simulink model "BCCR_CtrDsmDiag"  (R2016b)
settings: Solver=FixedStepDiscrete  StartTime=0.0  StopTime=10.0  FixedStep=0.02  RelTol=1e-3  EnableMultiTasking=on
undefined symbols (not defined in the file or in its folder): BCCR_cntDChrgCtrPlausDiag_CW, BCCR_cntMainCtrPlausDiag_CW, bin2dec
libraries: simulink x72

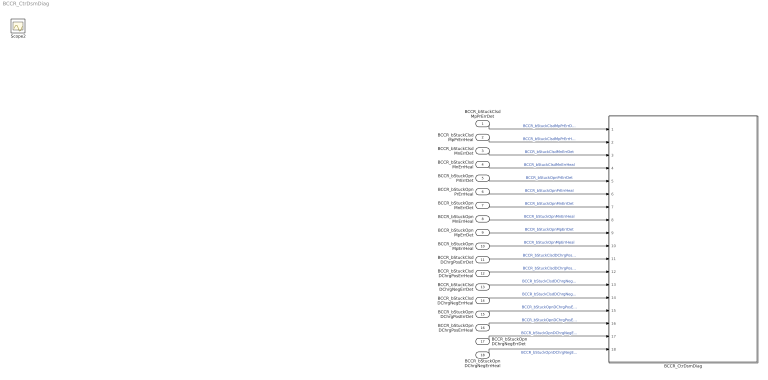
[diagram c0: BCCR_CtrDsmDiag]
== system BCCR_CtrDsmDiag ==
  BCCR_bStuckClsdMpPrErrDet : Inport
  BCCR_bStuckClsdMpPrErrHeal : Inport  Port=2
  BCCR_bStuckClsdMnErrDet : Inport  Port=3
  BCCR_bStuckClsdMnErrHeal : Inport  Port=4
  BCCR_bStuckOpnPrErrDet : Inport  Port=5
  BCCR_bStuckOpnPrErrHeal : Inport  Port=6
  BCCR_bStuckOpnMnErrDet : Inport  Port=7
  BCCR_bStuckOpnMnErrHeal : Inport  Port=8
  BCCR_bStuckOpnMpErrDet : Inport  Port=9
  BCCR_bStuckOpnMpErrHeal : Inport  Port=10
  BCCR_bStuckClsdDChrgPosErrDet : Inport  Port=11
  BCCR_bStuckClsdDChrgPosErrHeal : Inport  Port=12
  BCCR_bStuckClsdDChrgNegErrDet : Inport  Port=13
  BCCR_bStuckClsdDChrgNegErrHeal : Inport  Port=14
  BCCR_bStuckOpnDChrgPosErrDet : Inport  Port=15
  BCCR_bStuckOpnDChrgPosErrHeal : Inport  Port=16
  BCCR_bStuckOpnDChrgNegErrDet : Inport  Port=17
  BCCR_bStuckOpnDChrgNegErrHeal : Inport  Port=18
  BCCR_CtrDsmDiag : Subsystem
  Scope2 : Scope
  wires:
  BCCR_bStuckClsdMpPrErrDet/1 -> BCCR_CtrDsmDiag/1(BCCR_bStuckClsdMpPrErrDet)  "BCCR_bStuckClsdMpPrErrDet"
  BCCR_bStuckClsdMpPrErrHeal/1 -> BCCR_CtrDsmDiag/2(BCCR_bStuckClsdMpPrErrHeal)  "BCCR_bStuckClsdMpPrErrHeal"
  BCCR_bStuckClsdMnErrDet/1 -> BCCR_CtrDsmDiag/3(BCCR_bStuckClsdMnErrDet)  "BCCR_bStuckClsdMnErrDet"
  BCCR_bStuckClsdMnErrHeal/1 -> BCCR_CtrDsmDiag/4(BCCR_bStuckClsdMnErrHeal)  "BCCR_bStuckClsdMnErrHeal"
  BCCR_bStuckOpnPrErrDet/1 -> BCCR_CtrDsmDiag/5(BCCR_bStuckOpnPrErrDet)  "BCCR_bStuckOpnPrErrDet"
  BCCR_bStuckOpnPrErrHeal/1 -> BCCR_CtrDsmDiag/6(BCCR_bStuckOpnPrErrHeal)  "BCCR_bStuckOpnPrErrHeal"
  BCCR_bStuckOpnMnErrDet/1 -> BCCR_CtrDsmDiag/7(BCCR_bStuckOpnMnErrDet)  "BCCR_bStuckOpnMnErrDet"
  BCCR_bStuckOpnMnErrHeal/1 -> BCCR_CtrDsmDiag/8(BCCR_bStuckOpnMnErrHeal)  "BCCR_bStuckOpnMnErrHeal"
  BCCR_bStuckOpnMpErrDet/1 -> BCCR_CtrDsmDiag/9(BCCR_bStuckOpnMpErrDet)  "BCCR_bStuckOpnMpErrDet"
  BCCR_bStuckOpnMpErrHeal/1 -> BCCR_CtrDsmDiag/10(BCCR_bStuckOpnMpErrHeal)  "BCCR_bStuckOpnMpErrHeal"
  BCCR_bStuckClsdDChrgPosErrDet/1 -> BCCR_CtrDsmDiag/11(BCCR_bStuckClsdDChrgPosErrDet)  "BCCR_bStuckClsdDChrgPosErrDet"
  BCCR_bStuckClsdDChrgPosErrHeal/1 -> BCCR_CtrDsmDiag/12(BCCR_bStuckClsdDChrgPosErrHeal)  "BCCR_bStuckClsdDChrgPosErrHeal"
  BCCR_bStuckClsdDChrgNegErrDet/1 -> BCCR_CtrDsmDiag/13(BCCR_bStuckClsdDChrgNegErrDet)  "BCCR_bStuckClsdDChrgNegErrDet"
  BCCR_bStuckClsdDChrgNegErrHeal/1 -> BCCR_CtrDsmDiag/14(BCCR_bStuckClsdDChrgNegErrHeal)  "BCCR_bStuckClsdDChrgNegErrHeal"
  BCCR_bStuckOpnDChrgPosErrDet/1 -> BCCR_CtrDsmDiag/15(BCCR_bStuckOpnDChrgPosErrDet)  "BCCR_bStuckOpnDChrgPosErrDet"
  BCCR_bStuckOpnDChrgPosErrHeal/1 -> BCCR_CtrDsmDiag/16(BCCR_bStuckOpnDChrgPosErrHeal)  "BCCR_bStuckOpnDChrgPosErrHeal"
  BCCR_bStuckOpnDChrgNegErrDet/1 -> BCCR_CtrDsmDiag/17(BCCR_bStuckOpnDChrgNegErrDet)  "BCCR_bStuckOpnDChrgNegErrDet"
  BCCR_bStuckOpnDChrgNegErrHeal/1 -> BCCR_CtrDsmDiag/18(BCCR_bStuckOpnDChrgNegErrHeal)  "BCCR_bStuckOpnDChrgNegErrHeal"

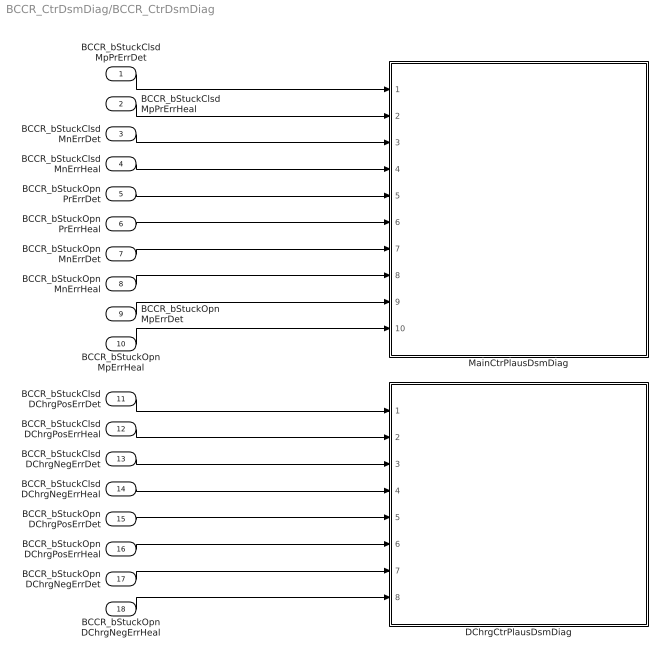
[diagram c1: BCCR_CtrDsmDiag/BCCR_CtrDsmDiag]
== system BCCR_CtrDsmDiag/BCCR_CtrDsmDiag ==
  BCCR_bStuckClsdMpPrErrDet : Inport
  BCCR_bStuckClsdMpPrErrHeal : Inport  Port=2
  BCCR_bStuckClsdMnErrDet : Inport  Port=3
  BCCR_bStuckClsdMnErrHeal : Inport  Port=4
  BCCR_bStuckOpnPrErrDet : Inport  Port=5
  BCCR_bStuckOpnPrErrHeal : Inport  Port=6
  BCCR_bStuckOpnMnErrDet : Inport  Port=7
  BCCR_bStuckOpnMnErrHeal : Inport  Port=8
  BCCR_bStuckOpnMpErrDet : Inport  Port=9
  BCCR_bStuckOpnMpErrHeal : Inport  Port=10
  BCCR_bStuckClsdDChrgPosErrDet : Inport  Port=11
  BCCR_bStuckClsdDChrgPosErrHeal : Inport  Port=12
  BCCR_bStuckClsdDChrgNegErrDet : Inport  Port=13
  BCCR_bStuckClsdDChrgNegErrHeal : Inport  Port=14
  BCCR_bStuckOpnDChrgPosErrDet : Inport  Port=15
  BCCR_bStuckOpnDChrgPosErrHeal : Inport  Port=16
  BCCR_bStuckOpnDChrgNegErrDet : Inport  Port=17
  BCCR_bStuckOpnDChrgNegErrHeal : Inport  Port=18
  DChrgCtrPlausDsmDiag : Subsystem
  MainCtrPlausDsmDiag : Subsystem
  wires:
  BCCR_bStuckClsdDChrgPosErrHeal/1 -> DChrgCtrPlausDsmDiag/2(BCCR_bStuckClsdDChrgPosErrHeal)
  BCCR_bStuckClsdDChrgNegErrHeal/1 -> DChrgCtrPlausDsmDiag/4(BCCR_bStuckClsdDChrgNegErrHeal)
  BCCR_bStuckOpnDChrgPosErrHeal/1 -> DChrgCtrPlausDsmDiag/6(BCCR_bStuckOpnDChrgPosErrHeal)
  BCCR_bStuckOpnDChrgNegErrDet/1 -> DChrgCtrPlausDsmDiag/7(BCCR_bStuckOpnDChrgNegErrDet)
  BCCR_bStuckOpnDChrgNegErrHeal/1 -> DChrgCtrPlausDsmDiag/8(BCCR_bStuckOpnDChrgNegErrHeal)
  BCCR_bStuckClsdMnErrDet/1 -> MainCtrPlausDsmDiag/3(BCCR_bStuckClsdMnErrDet)
  BCCR_bStuckClsdDChrgNegErrDet/1 -> DChrgCtrPlausDsmDiag/3(BCCR_bStuckClsdDChrgNegErrDet)
  BCCR_bStuckClsdMnErrHeal/1 -> MainCtrPlausDsmDiag/4(BCCR_bStuckClsdMnErrHeal)
  BCCR_bStuckClsdMpPrErrDet/1 -> MainCtrPlausDsmDiag/1(BCCR_bStuckClsdMpPrErrDet)
  BCCR_bStuckClsdMpPrErrHeal/1 -> MainCtrPlausDsmDiag/2(BCCR_bStuckClsdMpPrErrHeal)
  BCCR_bStuckClsdDChrgPosErrDet/1 -> DChrgCtrPlausDsmDiag/1(BCCR_bStuckClsdDChrgPosErrDet)
  BCCR_bStuckOpnDChrgPosErrDet/1 -> DChrgCtrPlausDsmDiag/5(BCCR_bStuckOpnDChrgPosErrDet)
  BCCR_bStuckOpnPrErrHeal/1 -> MainCtrPlausDsmDiag/6(BCCR_bStuckOpnPrErrHeal)
  BCCR_bStuckOpnMnErrDet/1 -> MainCtrPlausDsmDiag/7(BCCR_bStuckOpnMnErrDet)
  BCCR_bStuckOpnMpErrHeal/1 -> MainCtrPlausDsmDiag/10(BCCR_bStuckOpnMpErrHeal)
  BCCR_bStuckOpnPrErrDet/1 -> MainCtrPlausDsmDiag/5(BCCR_bStuckOpnPrErrDet)
  BCCR_bStuckOpnMpErrDet/1 -> MainCtrPlausDsmDiag/9(BCCR_bStuckOpnMpErrDet)
  BCCR_bStuckOpnMnErrHeal/1 -> MainCtrPlausDsmDiag/8(BCCR_bStuckOpnMnErrHeal)

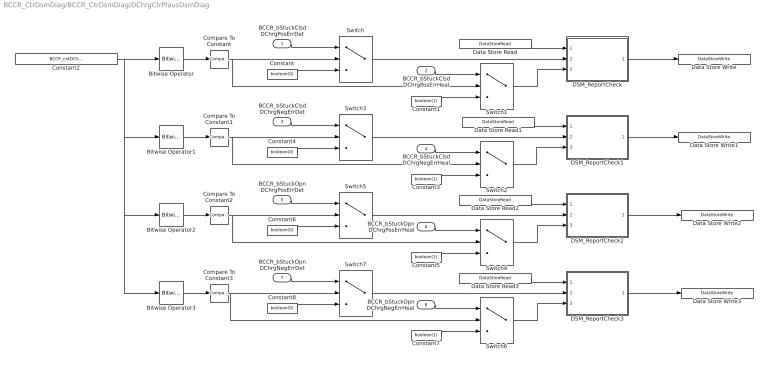
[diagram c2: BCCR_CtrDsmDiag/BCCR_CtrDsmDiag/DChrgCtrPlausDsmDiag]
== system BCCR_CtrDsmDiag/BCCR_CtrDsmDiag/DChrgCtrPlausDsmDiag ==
  BCCR_bStuckClsdDChrgPosErrDet : Inport
  BCCR_bStuckClsdDChrgPosErrHeal : Inport  Port=2
  BCCR_bStuckClsdDChrgNegErrDet : Inport  Port=3
  BCCR_bStuckClsdDChrgNegErrHeal : Inport  Port=4
  BCCR_bStuckOpnDChrgPosErrDet : Inport  Port=5
  BCCR_bStuckOpnDChrgPosErrHeal : Inport  Port=6
  BCCR_bStuckOpnDChrgNegErrDet : Inport  Port=7
  BCCR_bStuckOpnDChrgNegErrHeal : Inport  Port=8
  Bitwise Operator : simulink/Logic and Bit Operations/Bitwise Operator  logicop=AND  UseBitMask=on  BitMask=bin2dec('00000001')  BitMaskRealWorld=Stored Integer
  Bitwise Operator1 : simulink/Logic and Bit Operations/Bitwise Operator  logicop=AND  UseBitMask=on  BitMask=bin2dec('00000010')  BitMaskRealWorld=Stored Integer
  Bitwise Operator2 : simulink/Logic and Bit Operations/Bitwise Operator  logicop=AND  UseBitMask=on  BitMask=bin2dec('00000100')  BitMaskRealWorld=Stored Integer
  Bitwise Operator3 : simulink/Logic and Bit Operations/Bitwise Operator  logicop=AND  UseBitMask=on  BitMask=bin2dec('00001000')  BitMaskRealWorld=Stored Integer
  Compare To Constant : simulink/Logic and Bit Operations/Compare To Constant  relop===  const=1  OutDataTypeStr=boolean
  Compare To Constant1 : simulink/Logic and Bit Operations/Compare To Constant  relop===  const=2  OutDataTypeStr=boolean
  Compare To Constant2 : simulink/Logic and Bit Operations/Compare To Constant  relop===  const=4  OutDataTypeStr=boolean
  Compare To Constant3 : simulink/Logic and Bit Operations/Compare To Constant  relop===  const=8  OutDataTypeStr=boolean
  Constant{,4,6,8} (4 alike) : Constant  Value=boolean(0)  OutDataTypeStr=boolean
  Constant{1,3,5,7} (4 alike) : Constant  Value=boolean(1)  OutDataTypeStr=boolean
  Constant2 : Constant  Value=BCCR_cntDChrgCtrPlausDiag_CW
  DSM_ReportCheck : Subsystem  TreatAsAtomicUnit=on  RTWFcnName=DSM_ReportCheck  RTWFileName=SrvLib
  DSM_ReportCheck1 : Subsystem  TreatAsAtomicUnit=on  RTWFcnName=DSM_ReportCheck  RTWFileName=SrvLib
  DSM_ReportCheck2 : Subsystem  TreatAsAtomicUnit=on  RTWFcnName=DSM_ReportCheck  RTWFileName=SrvLib
  DSM_ReportCheck3 : Subsystem  TreatAsAtomicUnit=on  RTWFcnName=DSM_ReportCheck  RTWFileName=SrvLib
  Data Store Read : DataStoreRead  DataStoreName=DFC_DChrgPosStuckMax
  Data Store Read1 : DataStoreRead  DataStoreName=DFC_DChrgNegStuckMax
  Data Store Read2 : DataStoreRead  DataStoreName=DFC_DChrgPosStuckMin
  Data Store Read3 : DataStoreRead  DataStoreName=DFC_DChrgNegStuckMin
  Data Store Write : DataStoreWrite  DataStoreName=DFC_DChrgPosStuckMax
  Data Store Write1 : DataStoreWrite  DataStoreName=DFC_DChrgNegStuckMax
  Data Store Write2 : DataStoreWrite  DataStoreName=DFC_DChrgPosStuckMin
  Data Store Write3 : DataStoreWrite  DataStoreName=DFC_DChrgNegStuckMin
  Switch{,1..7} (8 alike) : Switch  Criteria=u2 > Threshold
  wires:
  DSM_ReportCheck/1(Dfc_id) -> Data Store Write/1
  DSM_ReportCheck1/1(Dfc_id) -> Data Store Write1/1
  Data Store Read2/1 -> DSM_ReportCheck2/1(Dfc_id_nv)
  Data Store Read/1 -> DSM_ReportCheck/1(Dfc_id_nv)
  DSM_ReportCheck2/1(Dfc_id) -> Data Store Write2/1
  Data Store Read3/1 -> DSM_ReportCheck3/1(Dfc_id_nv)
  Data Store Read1/1 -> DSM_ReportCheck1/1(Dfc_id_nv)
  DSM_ReportCheck3/1(Dfc_id) -> Data Store Write3/1
  Constant/1 -> Switch/3
  BCCR_bStuckClsdDChrgPosErrHeal/1 -> Switch1/1
  Constant1/1 -> Switch1/3
  Switch1/1 -> DSM_ReportCheck/3(Heal)
  Switch/1 -> DSM_ReportCheck/2(Err)
  Bitwise Operator/1 -> Compare To Constant/1
  Compare To Constant/1 -> Switch/2, Switch1/2
  BCCR_bStuckClsdDChrgPosErrDet/1 -> Switch/1
  Constant3/1 -> Switch2/3
  Constant4/1 -> Switch3/3
  Switch3/1 -> DSM_ReportCheck1/2(Err)
  Switch2/1 -> DSM_ReportCheck1/3(Heal)
  BCCR_bStuckClsdDChrgNegErrHeal/1 -> Switch2/1
  BCCR_bStuckClsdDChrgNegErrDet/1 -> Switch3/1
  Constant2/1 -> Bitwise Operator3/1, Bitwise Operator2/1, Bitwise Operator1/1, Bitwise Operator/1
  Bitwise Operator1/1 -> Compare To Constant1/1
  Compare To Constant1/1 -> Switch2/2, Switch3/2
  Constant5/1 -> Switch4/3
  Switch4/1 -> DSM_ReportCheck2/3(Heal)
  Constant6/1 -> Switch5/3
  Switch5/1 -> DSM_ReportCheck2/2(Err)
  BCCR_bStuckOpnDChrgPosErrHeal/1 -> Switch4/1
  BCCR_bStuckOpnDChrgPosErrDet/1 -> Switch5/1
  Bitwise Operator2/1 -> Compare To Constant2/1
  Compare To Constant2/1 -> Switch4/2, Switch5/2
  Constant7/1 -> Switch6/3
  Switch6/1 -> DSM_ReportCheck3/3(Heal)
  Constant8/1 -> Switch7/3
  Switch7/1 -> DSM_ReportCheck3/2(Err)
  BCCR_bStuckOpnDChrgNegErrHeal/1 -> Switch6/1
  BCCR_bStuckOpnDChrgNegErrDet/1 -> Switch7/1
  Bitwise Operator3/1 -> Compare To Constant3/1
  Compare To Constant3/1 -> Switch6/2, Switch7/2

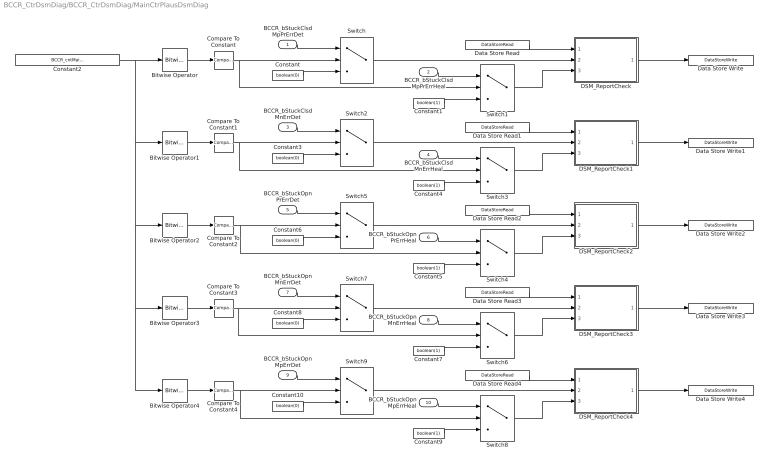
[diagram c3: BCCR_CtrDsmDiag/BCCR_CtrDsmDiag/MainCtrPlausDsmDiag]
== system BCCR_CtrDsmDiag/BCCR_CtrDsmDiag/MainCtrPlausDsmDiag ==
  BCCR_bStuckClsdMpPrErrDet : Inport
  BCCR_bStuckClsdMpPrErrHeal : Inport  Port=2
  BCCR_bStuckClsdMnErrDet : Inport  Port=3
  BCCR_bStuckClsdMnErrHeal : Inport  Port=4
  BCCR_bStuckOpnPrErrDet : Inport  Port=5
  BCCR_bStuckOpnPrErrHeal : Inport  Port=6
  BCCR_bStuckOpnMnErrDet : Inport  Port=7
  BCCR_bStuckOpnMnErrHeal : Inport  Port=8
  BCCR_bStuckOpnMpErrDet : Inport  Port=9
  BCCR_bStuckOpnMpErrHeal : Inport  Port=10
  Bitwise Operator : simulink/Logic and Bit Operations/Bitwise Operator  logicop=AND  UseBitMask=on  BitMask=bin2dec('00000001')  BitMaskRealWorld=Stored Integer
  Bitwise Operator1 : simulink/Logic and Bit Operations/Bitwise Operator  logicop=AND  UseBitMask=on  BitMask=bin2dec('00000010')  BitMaskRealWorld=Stored Integer
  Bitwise Operator2 : simulink/Logic and Bit Operations/Bitwise Operator  logicop=AND  UseBitMask=on  BitMask=bin2dec('00000100')  BitMaskRealWorld=Stored Integer
  Bitwise Operator3 : simulink/Logic and Bit Operations/Bitwise Operator  logicop=AND  UseBitMask=on  BitMask=bin2dec('00001000')  BitMaskRealWorld=Stored Integer
  Bitwise Operator4 : simulink/Logic and Bit Operations/Bitwise Operator  logicop=AND  UseBitMask=on  BitMask=bin2dec('00010000')  BitMaskRealWorld=Stored Integer
  Compare To Constant : simulink/Logic and Bit Operations/Compare To Constant  relop===  const=1  OutDataTypeStr=boolean
  Compare To Constant1 : simulink/Logic and Bit Operations/Compare To Constant  relop===  const=2  OutDataTypeStr=boolean
  Compare To Constant2 : simulink/Logic and Bit Operations/Compare To Constant  relop===  const=4  OutDataTypeStr=boolean
  Compare To Constant3 : simulink/Logic and Bit Operations/Compare To Constant  relop===  const=8  OutDataTypeStr=boolean
  Compare To Constant4 : simulink/Logic and Bit Operations/Compare To Constant  relop===  const=16  OutDataTypeStr=boolean
  Constant{,3,6,8,10} (5 alike) : Constant  Value=boolean(0)  OutDataTypeStr=boolean
  Constant{1,4..5,7,9} (5 alike) : Constant  Value=boolean(1)  OutDataTypeStr=boolean
  Constant2 : Constant  Value=BCCR_cntMainCtrPlausDiag_CW
  DSM_ReportCheck : Subsystem  TreatAsAtomicUnit=on  RTWFcnName=DSM_ReportCheck  RTWFileName=SrvLib
  DSM_ReportCheck1 : Subsystem  TreatAsAtomicUnit=on  RTWFcnName=DSM_ReportCheck  RTWFileName=SrvLib
  DSM_ReportCheck2 : Subsystem  TreatAsAtomicUnit=on  RTWFcnName=DSM_ReportCheck  RTWFileName=SrvLib
  DSM_ReportCheck3 : Subsystem  TreatAsAtomicUnit=on  RTWFcnName=DSM_ReportCheck  RTWFileName=SrvLib
  DSM_ReportCheck4 : Subsystem  TreatAsAtomicUnit=on  RTWFcnName=DSM_ReportCheck  RTWFileName=SrvLib
  Data Store Read : DataStoreRead  DataStoreName=DFC_PosStuckMax
  Data Store Read1 : DataStoreRead  DataStoreName=DFC_MNegStuckMax
  Data Store Read2 : DataStoreRead  DataStoreName=DFC_PrStuckMin
  Data Store Read3 : DataStoreRead  DataStoreName=DFC_MNegStuckMin
  Data Store Read4 : DataStoreRead  DataStoreName=DFC_MPosStuckMin
  Data Store Write : DataStoreWrite  DataStoreName=DFC_PosStuckMax
  Data Store Write1 : DataStoreWrite  DataStoreName=DFC_MNegStuckMax
  Data Store Write2 : DataStoreWrite  DataStoreName=DFC_PrStuckMin
  Data Store Write3 : DataStoreWrite  DataStoreName=DFC_MNegStuckMin
  Data Store Write4 : DataStoreWrite  DataStoreName=DFC_MPosStuckMin
  Switch{,1..9} (10 alike) : Switch  Criteria=u2 > Threshold
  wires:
  Data Store Read4/1 -> DSM_ReportCheck4/1(Dfc_id_nv)
  DSM_ReportCheck3/1(Dfc_id) -> Data Store Write3/1
  Data Store Read1/1 -> DSM_ReportCheck1/1(Dfc_id_nv)
  Data Store Read3/1 -> DSM_ReportCheck3/1(Dfc_id_nv)
  DSM_ReportCheck2/1(Dfc_id) -> Data Store Write2/1
  Data Store Read/1 -> DSM_ReportCheck/1(Dfc_id_nv)
  Data Store Read2/1 -> DSM_ReportCheck2/1(Dfc_id_nv)
  DSM_ReportCheck1/1(Dfc_id) -> Data Store Write1/1
  DSM_ReportCheck/1(Dfc_id) -> Data Store Write/1
  DSM_ReportCheck4/1(Dfc_id) -> Data Store Write4/1
  Constant/1 -> Switch/3
  BCCR_bStuckClsdMpPrErrDet/1 -> Switch/1
  BCCR_bStuckClsdMpPrErrHeal/1 -> Switch1/1
  Constant1/1 -> Switch1/3
  Switch1/1 -> DSM_ReportCheck/3(Heal)
  Switch/1 -> DSM_ReportCheck/2(Err)
  Constant2/1 -> Bitwise Operator3/1, Bitwise Operator4/1, Bitwise Operator2/1, Bitwise Operator1/1, Bitwise Operator/1
  Bitwise Operator/1 -> Compare To Constant/1
  Compare To Constant/1 -> Switch1/2, Switch/2
  Constant3/1 -> Switch2/3
  Constant4/1 -> Switch3/3
  Switch3/1 -> DSM_ReportCheck1/3(Heal)
  Switch2/1 -> DSM_ReportCheck1/2(Err)
  BCCR_bStuckClsdMnErrHeal/1 -> Switch3/1
  BCCR_bStuckClsdMnErrDet/1 -> Switch2/1
  Bitwise Operator1/1 -> Compare To Constant1/1
  Compare To Constant1/1 -> Switch3/2, Switch2/2
  Constant5/1 -> Switch4/3
  Switch4/1 -> DSM_ReportCheck2/3(Heal)
  Constant6/1 -> Switch5/3
  Switch5/1 -> DSM_ReportCheck2/2(Err)
  BCCR_bStuckOpnPrErrHeal/1 -> Switch4/1
  BCCR_bStuckOpnPrErrDet/1 -> Switch5/1
  Bitwise Operator2/1 -> Compare To Constant2/1
  Compare To Constant2/1 -> Switch4/2, Switch5/2
  Constant7/1 -> Switch6/3
  Switch6/1 -> DSM_ReportCheck3/3(Heal)
  Constant8/1 -> Switch7/3
  Switch7/1 -> DSM_ReportCheck3/2(Err)
  Bitwise Operator3/1 -> Compare To Constant3/1
  Compare To Constant3/1 -> Switch6/2, Switch7/2
  BCCR_bStuckOpnMnErrDet/1 -> Switch7/1
  BCCR_bStuckOpnMnErrHeal/1 -> Switch6/1
  Constant9/1 -> Switch8/3
  Constant10/1 -> Switch9/3
  Switch9/1 -> DSM_ReportCheck4/2(Err)
  Switch8/1 -> DSM_ReportCheck4/3(Heal)
  BCCR_bStuckOpnMpErrHeal/1 -> Switch8/1
  BCCR_bStuckOpnMpErrDet/1 -> Switch9/1
  Bitwise Operator4/1 -> Compare To Constant4/1
  Compare To Constant4/1 -> Switch8/2, Switch9/2

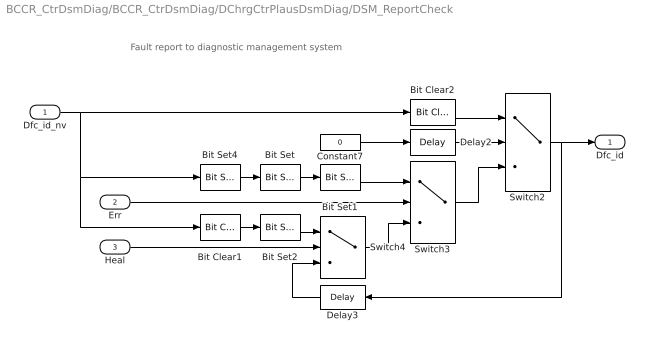
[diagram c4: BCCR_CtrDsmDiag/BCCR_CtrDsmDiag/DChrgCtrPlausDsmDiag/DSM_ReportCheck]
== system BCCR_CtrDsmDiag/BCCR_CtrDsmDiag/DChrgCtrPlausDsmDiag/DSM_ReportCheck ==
  note: Fault report to diagnostic management system
  Dfc_id_nv : Inport  OutDataTypeStr=uint8
  Err : Inport  Port=2
  Heal : Inport  Port=3
  Bit Clear1 : simulink/Logic and Bit Operations/Bit Clear  iBit=4
  Bit Clear2 : simulink/Logic and Bit Operations/Bit Clear  iBit=3
  Bit Set : simulink/Logic and Bit Operations/Bit Set  iBit=4
  Bit Set1 : simulink/Logic and Bit Operations/Bit Set  iBit=3
  Bit Set2 : simulink/Logic and Bit Operations/Bit Set  iBit=3
  Bit Set4 : simulink/Logic and Bit Operations/Bit Set  iBit=7
  Constant7 : Constant  Value=0  OutDataTypeStr=boolean
  Delay2 : Delay  DelayLength=1  InitialCondition=1
  Delay3 : Delay  DelayLength=1  InitialCondition=0
  Switch2 : Switch  Criteria=u2 ~= 0
  Switch3 : Switch  Criteria=u2 ~= 0
  Switch4 : Switch  Criteria=u2 ~= 0
  Dfc_id : Outport  OutDataTypeStr=uint8
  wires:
  Dfc_id_nv/1 -> Bit Clear2/1, Bit Set4/1, Bit Clear1/1
  Bit Set4/1 -> Bit Set/1
  Constant7/1 -> Delay2/1
  Delay2/1 -> Switch2/2
  Switch3/1 -> Switch2/3
  Bit Clear2/1 -> Switch2/1
  Switch2/1 -> Delay3/1, Dfc_id/1
  Bit Set1/1 -> Switch3/1
  Bit Set/1 -> Bit Set1/1
  Switch4/1 -> Switch3/3
  Err/1 -> Switch3/2
  Bit Set2/1 -> Switch4/1
  Bit Clear1/1 -> Bit Set2/1
  Delay3/1 -> Switch4/3
  Heal/1 -> Switch4/2

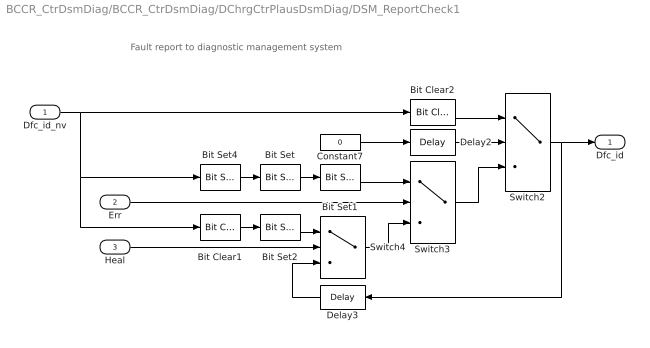
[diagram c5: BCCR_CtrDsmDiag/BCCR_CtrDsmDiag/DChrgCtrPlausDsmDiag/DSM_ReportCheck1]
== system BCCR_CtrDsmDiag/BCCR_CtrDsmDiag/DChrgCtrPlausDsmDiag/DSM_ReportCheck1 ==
  note: Fault report to diagnostic management system
  Dfc_id_nv : Inport  OutDataTypeStr=uint8
  Err : Inport  Port=2
  Heal : Inport  Port=3
  Bit Clear1 : simulink/Logic and Bit Operations/Bit Clear  iBit=4
  Bit Clear2 : simulink/Logic and Bit Operations/Bit Clear  iBit=3
  Bit Set : simulink/Logic and Bit Operations/Bit Set  iBit=4
  Bit Set1 : simulink/Logic and Bit Operations/Bit Set  iBit=3
  Bit Set2 : simulink/Logic and Bit Operations/Bit Set  iBit=3
  Bit Set4 : simulink/Logic and Bit Operations/Bit Set  iBit=7
  Constant7 : Constant  Value=0  OutDataTypeStr=boolean
  Delay2 : Delay  DelayLength=1  InitialCondition=1
  Delay3 : Delay  DelayLength=1  InitialCondition=0
  Switch2 : Switch  Criteria=u2 ~= 0
  Switch3 : Switch  Criteria=u2 ~= 0
  Switch4 : Switch  Criteria=u2 ~= 0
  Dfc_id : Outport  OutDataTypeStr=uint8
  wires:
  Heal/1 -> Switch4/2
  Delay3/1 -> Switch4/3
  Bit Clear1/1 -> Bit Set2/1
  Bit Set2/1 -> Switch4/1
  Err/1 -> Switch3/2
  Switch4/1 -> Switch3/3
  Bit Set/1 -> Bit Set1/1
  Bit Set1/1 -> Switch3/1
  Switch2/1 -> Dfc_id/1, Delay3/1
  Bit Clear2/1 -> Switch2/1
  Switch3/1 -> Switch2/3
  Delay2/1 -> Switch2/2
  Constant7/1 -> Delay2/1
  Bit Set4/1 -> Bit Set/1
  Dfc_id_nv/1 -> Bit Clear1/1, Bit Set4/1, Bit Clear2/1

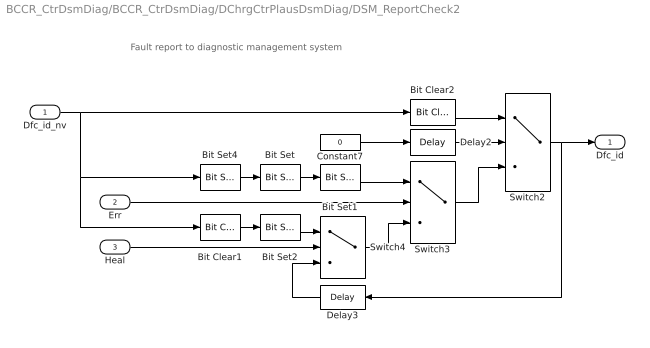
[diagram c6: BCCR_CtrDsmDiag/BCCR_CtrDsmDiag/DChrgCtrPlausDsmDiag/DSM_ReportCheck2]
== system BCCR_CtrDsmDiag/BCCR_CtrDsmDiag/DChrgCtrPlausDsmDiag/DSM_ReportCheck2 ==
  note: Fault report to diagnostic management system
  Dfc_id_nv : Inport  OutDataTypeStr=uint8
  Err : Inport  Port=2
  Heal : Inport  Port=3
  Bit Clear1 : simulink/Logic and Bit Operations/Bit Clear  iBit=4
  Bit Clear2 : simulink/Logic and Bit Operations/Bit Clear  iBit=3
  Bit Set : simulink/Logic and Bit Operations/Bit Set  iBit=4
  Bit Set1 : simulink/Logic and Bit Operations/Bit Set  iBit=3
  Bit Set2 : simulink/Logic and Bit Operations/Bit Set  iBit=3
  Bit Set4 : simulink/Logic and Bit Operations/Bit Set  iBit=7
  Constant7 : Constant  Value=0  OutDataTypeStr=boolean
  Delay2 : Delay  DelayLength=1  InitialCondition=1
  Delay3 : Delay  DelayLength=1  InitialCondition=0
  Switch2 : Switch  Criteria=u2 ~= 0
  Switch3 : Switch  Criteria=u2 ~= 0
  Switch4 : Switch  Criteria=u2 ~= 0
  Dfc_id : Outport  OutDataTypeStr=uint8
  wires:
  Dfc_id_nv/1 -> Bit Clear2/1, Bit Set4/1, Bit Clear1/1
  Bit Set4/1 -> Bit Set/1
  Constant7/1 -> Delay2/1
  Delay2/1 -> Switch2/2
  Switch3/1 -> Switch2/3
  Bit Clear2/1 -> Switch2/1
  Switch2/1 -> Delay3/1, Dfc_id/1
  Bit Set1/1 -> Switch3/1
  Bit Set/1 -> Bit Set1/1
  Switch4/1 -> Switch3/3
  Err/1 -> Switch3/2
  Bit Set2/1 -> Switch4/1
  Bit Clear1/1 -> Bit Set2/1
  Delay3/1 -> Switch4/3
  Heal/1 -> Switch4/2

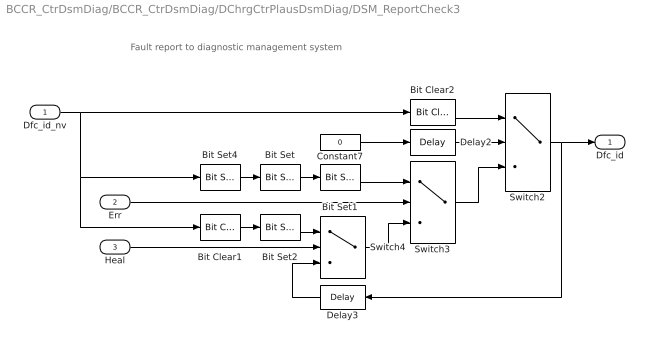
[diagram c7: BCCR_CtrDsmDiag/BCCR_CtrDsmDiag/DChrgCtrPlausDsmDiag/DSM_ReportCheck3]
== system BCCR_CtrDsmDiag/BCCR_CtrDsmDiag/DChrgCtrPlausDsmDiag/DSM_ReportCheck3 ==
  note: Fault report to diagnostic management system
  Dfc_id_nv : Inport  OutDataTypeStr=uint8
  Err : Inport  Port=2
  Heal : Inport  Port=3
  Bit Clear1 : simulink/Logic and Bit Operations/Bit Clear  iBit=4
  Bit Clear2 : simulink/Logic and Bit Operations/Bit Clear  iBit=3
  Bit Set : simulink/Logic and Bit Operations/Bit Set  iBit=4
  Bit Set1 : simulink/Logic and Bit Operations/Bit Set  iBit=3
  Bit Set2 : simulink/Logic and Bit Operations/Bit Set  iBit=3
  Bit Set4 : simulink/Logic and Bit Operations/Bit Set  iBit=7
  Constant7 : Constant  Value=0  OutDataTypeStr=boolean
  Delay2 : Delay  DelayLength=1  InitialCondition=1
  Delay3 : Delay  DelayLength=1  InitialCondition=0
  Switch2 : Switch  Criteria=u2 ~= 0
  Switch3 : Switch  Criteria=u2 ~= 0
  Switch4 : Switch  Criteria=u2 ~= 0
  Dfc_id : Outport  OutDataTypeStr=uint8
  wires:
  Heal/1 -> Switch4/2
  Delay3/1 -> Switch4/3
  Bit Clear1/1 -> Bit Set2/1
  Bit Set2/1 -> Switch4/1
  Err/1 -> Switch3/2
  Switch4/1 -> Switch3/3
  Bit Set/1 -> Bit Set1/1
  Bit Set1/1 -> Switch3/1
  Switch2/1 -> Dfc_id/1, Delay3/1
  Bit Clear2/1 -> Switch2/1
  Switch3/1 -> Switch2/3
  Delay2/1 -> Switch2/2
  Constant7/1 -> Delay2/1
  Bit Set4/1 -> Bit Set/1
  Dfc_id_nv/1 -> Bit Clear1/1, Bit Set4/1, Bit Clear2/1

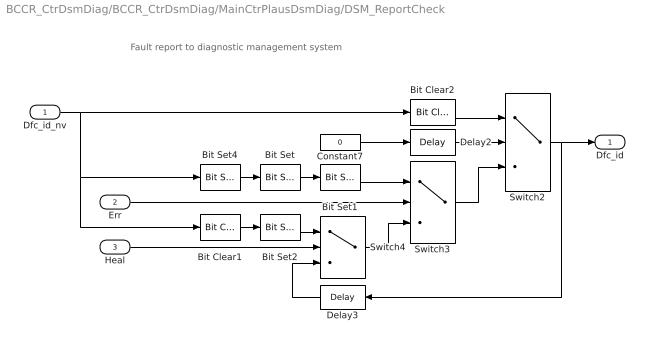
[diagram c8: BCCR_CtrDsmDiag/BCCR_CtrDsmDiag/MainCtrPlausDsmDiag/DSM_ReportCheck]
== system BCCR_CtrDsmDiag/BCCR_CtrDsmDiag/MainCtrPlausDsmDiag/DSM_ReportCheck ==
  note: Fault report to diagnostic management system
  Dfc_id_nv : Inport  OutDataTypeStr=uint8
  Err : Inport  Port=2
  Heal : Inport  Port=3
  Bit Clear1 : simulink/Logic and Bit Operations/Bit Clear  iBit=4
  Bit Clear2 : simulink/Logic and Bit Operations/Bit Clear  iBit=3
  Bit Set : simulink/Logic and Bit Operations/Bit Set  iBit=4
  Bit Set1 : simulink/Logic and Bit Operations/Bit Set  iBit=3
  Bit Set2 : simulink/Logic and Bit Operations/Bit Set  iBit=3
  Bit Set4 : simulink/Logic and Bit Operations/Bit Set  iBit=7
  Constant7 : Constant  Value=0  OutDataTypeStr=boolean
  Delay2 : Delay  DelayLength=1  InitialCondition=1
  Delay3 : Delay  DelayLength=1  InitialCondition=0
  Switch2 : Switch  Criteria=u2 ~= 0
  Switch3 : Switch  Criteria=u2 ~= 0
  Switch4 : Switch  Criteria=u2 ~= 0
  Dfc_id : Outport  OutDataTypeStr=uint8
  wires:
  Dfc_id_nv/1 -> Bit Clear2/1, Bit Set4/1, Bit Clear1/1
  Bit Set4/1 -> Bit Set/1
  Constant7/1 -> Delay2/1
  Delay2/1 -> Switch2/2
  Switch3/1 -> Switch2/3
  Bit Clear2/1 -> Switch2/1
  Switch2/1 -> Delay3/1, Dfc_id/1
  Bit Set1/1 -> Switch3/1
  Bit Set/1 -> Bit Set1/1
  Switch4/1 -> Switch3/3
  Err/1 -> Switch3/2
  Bit Set2/1 -> Switch4/1
  Bit Clear1/1 -> Bit Set2/1
  Delay3/1 -> Switch4/3
  Heal/1 -> Switch4/2

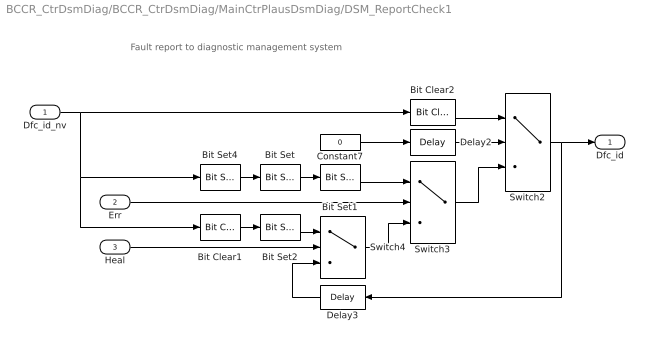
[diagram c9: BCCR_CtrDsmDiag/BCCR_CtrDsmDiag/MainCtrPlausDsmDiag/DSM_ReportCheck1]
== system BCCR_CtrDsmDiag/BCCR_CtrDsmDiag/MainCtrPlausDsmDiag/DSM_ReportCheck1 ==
  note: Fault report to diagnostic management system
  Dfc_id_nv : Inport  OutDataTypeStr=uint8
  Err : Inport  Port=2
  Heal : Inport  Port=3
  Bit Clear1 : simulink/Logic and Bit Operations/Bit Clear  iBit=4
  Bit Clear2 : simulink/Logic and Bit Operations/Bit Clear  iBit=3
  Bit Set : simulink/Logic and Bit Operations/Bit Set  iBit=4
  Bit Set1 : simulink/Logic and Bit Operations/Bit Set  iBit=3
  Bit Set2 : simulink/Logic and Bit Operations/Bit Set  iBit=3
  Bit Set4 : simulink/Logic and Bit Operations/Bit Set  iBit=7
  Constant7 : Constant  Value=0  OutDataTypeStr=boolean
  Delay2 : Delay  DelayLength=1  InitialCondition=1
  Delay3 : Delay  DelayLength=1  InitialCondition=0
  Switch2 : Switch  Criteria=u2 ~= 0
  Switch3 : Switch  Criteria=u2 ~= 0
  Switch4 : Switch  Criteria=u2 ~= 0
  Dfc_id : Outport  OutDataTypeStr=uint8
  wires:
  Heal/1 -> Switch4/2
  Delay3/1 -> Switch4/3
  Bit Clear1/1 -> Bit Set2/1
  Bit Set2/1 -> Switch4/1
  Err/1 -> Switch3/2
  Switch4/1 -> Switch3/3
  Bit Set/1 -> Bit Set1/1
  Bit Set1/1 -> Switch3/1
  Switch2/1 -> Dfc_id/1, Delay3/1
  Bit Clear2/1 -> Switch2/1
  Switch3/1 -> Switch2/3
  Delay2/1 -> Switch2/2
  Constant7/1 -> Delay2/1
  Bit Set4/1 -> Bit Set/1
  Dfc_id_nv/1 -> Bit Clear1/1, Bit Set4/1, Bit Clear2/1

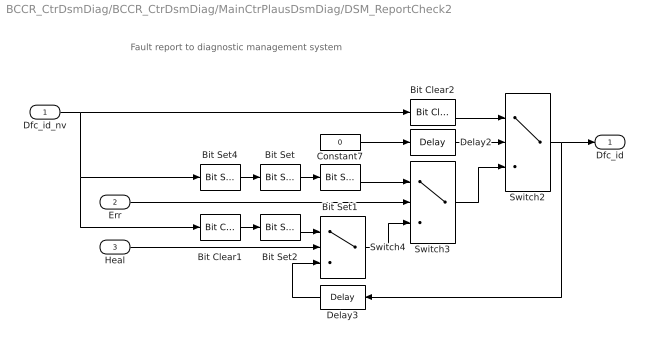
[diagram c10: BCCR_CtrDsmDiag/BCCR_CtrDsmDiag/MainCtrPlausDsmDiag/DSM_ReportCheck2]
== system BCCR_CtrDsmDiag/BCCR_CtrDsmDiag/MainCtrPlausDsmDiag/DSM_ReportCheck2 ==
  note: Fault report to diagnostic management system
  Dfc_id_nv : Inport  OutDataTypeStr=uint8
  Err : Inport  Port=2
  Heal : Inport  Port=3
  Bit Clear1 : simulink/Logic and Bit Operations/Bit Clear  iBit=4
  Bit Clear2 : simulink/Logic and Bit Operations/Bit Clear  iBit=3
  Bit Set : simulink/Logic and Bit Operations/Bit Set  iBit=4
  Bit Set1 : simulink/Logic and Bit Operations/Bit Set  iBit=3
  Bit Set2 : simulink/Logic and Bit Operations/Bit Set  iBit=3
  Bit Set4 : simulink/Logic and Bit Operations/Bit Set  iBit=7
  Constant7 : Constant  Value=0  OutDataTypeStr=boolean
  Delay2 : Delay  DelayLength=1  InitialCondition=1
  Delay3 : Delay  DelayLength=1  InitialCondition=0
  Switch2 : Switch  Criteria=u2 ~= 0
  Switch3 : Switch  Criteria=u2 ~= 0
  Switch4 : Switch  Criteria=u2 ~= 0
  Dfc_id : Outport  OutDataTypeStr=uint8
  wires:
  Dfc_id_nv/1 -> Bit Clear2/1, Bit Set4/1, Bit Clear1/1
  Bit Set4/1 -> Bit Set/1
  Constant7/1 -> Delay2/1
  Delay2/1 -> Switch2/2
  Switch3/1 -> Switch2/3
  Bit Clear2/1 -> Switch2/1
  Switch2/1 -> Delay3/1, Dfc_id/1
  Bit Set1/1 -> Switch3/1
  Bit Set/1 -> Bit Set1/1
  Switch4/1 -> Switch3/3
  Err/1 -> Switch3/2
  Bit Set2/1 -> Switch4/1
  Bit Clear1/1 -> Bit Set2/1
  Delay3/1 -> Switch4/3
  Heal/1 -> Switch4/2

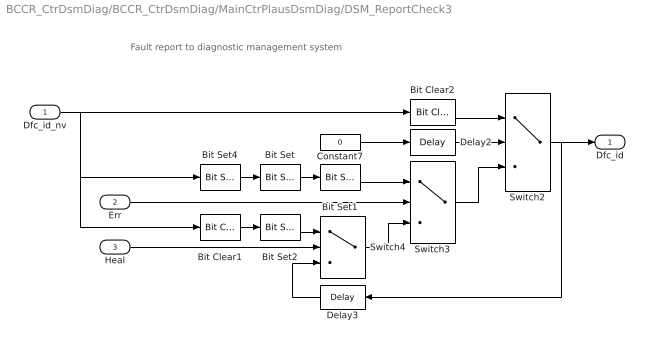
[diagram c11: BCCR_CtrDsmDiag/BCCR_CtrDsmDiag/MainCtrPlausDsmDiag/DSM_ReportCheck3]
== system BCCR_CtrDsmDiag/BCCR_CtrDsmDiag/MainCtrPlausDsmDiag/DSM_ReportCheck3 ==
  note: Fault report to diagnostic management system
  Dfc_id_nv : Inport  OutDataTypeStr=uint8
  Err : Inport  Port=2
  Heal : Inport  Port=3
  Bit Clear1 : simulink/Logic and Bit Operations/Bit Clear  iBit=4
  Bit Clear2 : simulink/Logic and Bit Operations/Bit Clear  iBit=3
  Bit Set : simulink/Logic and Bit Operations/Bit Set  iBit=4
  Bit Set1 : simulink/Logic and Bit Operations/Bit Set  iBit=3
  Bit Set2 : simulink/Logic and Bit Operations/Bit Set  iBit=3
  Bit Set4 : simulink/Logic and Bit Operations/Bit Set  iBit=7
  Constant7 : Constant  Value=0  OutDataTypeStr=boolean
  Delay2 : Delay  DelayLength=1  InitialCondition=1
  Delay3 : Delay  DelayLength=1  InitialCondition=0
  Switch2 : Switch  Criteria=u2 ~= 0
  Switch3 : Switch  Criteria=u2 ~= 0
  Switch4 : Switch  Criteria=u2 ~= 0
  Dfc_id : Outport  OutDataTypeStr=uint8
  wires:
  Heal/1 -> Switch4/2
  Delay3/1 -> Switch4/3
  Bit Clear1/1 -> Bit Set2/1
  Bit Set2/1 -> Switch4/1
  Err/1 -> Switch3/2
  Switch4/1 -> Switch3/3
  Bit Set/1 -> Bit Set1/1
  Bit Set1/1 -> Switch3/1
  Switch2/1 -> Dfc_id/1, Delay3/1
  Bit Clear2/1 -> Switch2/1
  Switch3/1 -> Switch2/3
  Delay2/1 -> Switch2/2
  Constant7/1 -> Delay2/1
  Bit Set4/1 -> Bit Set/1
  Dfc_id_nv/1 -> Bit Clear1/1, Bit Set4/1, Bit Clear2/1

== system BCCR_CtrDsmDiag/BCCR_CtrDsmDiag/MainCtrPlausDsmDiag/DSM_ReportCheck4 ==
  note: Fault report to diagnostic management system
  Dfc_id_nv : Inport  OutDataTypeStr=uint8
  Err : Inport  Port=2
  Heal : Inport  Port=3
  Bit Clear1 : simulink/Logic and Bit Operations/Bit Clear  iBit=4
  Bit Clear2 : simulink/Logic and Bit Operations/Bit Clear  iBit=3
  Bit Set : simulink/Logic and Bit Operations/Bit Set  iBit=4
  Bit Set1 : simulink/Logic and Bit Operations/Bit Set  iBit=3
  Bit Set2 : simulink/Logic and Bit Operations/Bit Set  iBit=3
  Bit Set4 : simulink/Logic and Bit Operations/Bit Set  iBit=7
  Constant7 : Constant  Value=0  OutDataTypeStr=boolean
  Delay2 : Delay  DelayLength=1  InitialCondition=1
  Delay3 : Delay  DelayLength=1  InitialCondition=0
  Switch2 : Switch  Criteria=u2 ~= 0
  Switch3 : Switch  Criteria=u2 ~= 0
  Switch4 : Switch  Criteria=u2 ~= 0
  Dfc_id : Outport  OutDataTypeStr=uint8
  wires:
  Dfc_id_nv/1 -> Bit Clear2/1, Bit Set4/1, Bit Clear1/1
  Bit Set4/1 -> Bit Set/1
  Constant7/1 -> Delay2/1
  Delay2/1 -> Switch2/2
  Switch3/1 -> Switch2/3
  Bit Clear2/1 -> Switch2/1
  Switch2/1 -> Delay3/1, Dfc_id/1
  Bit Set1/1 -> Switch3/1
  Bit Set/1 -> Bit Set1/1
  Switch4/1 -> Switch3/3
  Err/1 -> Switch3/2
  Bit Set2/1 -> Switch4/1
  Bit Clear1/1 -> Bit Set2/1
  Delay3/1 -> Switch4/3
  Heal/1 -> Switch4/2
